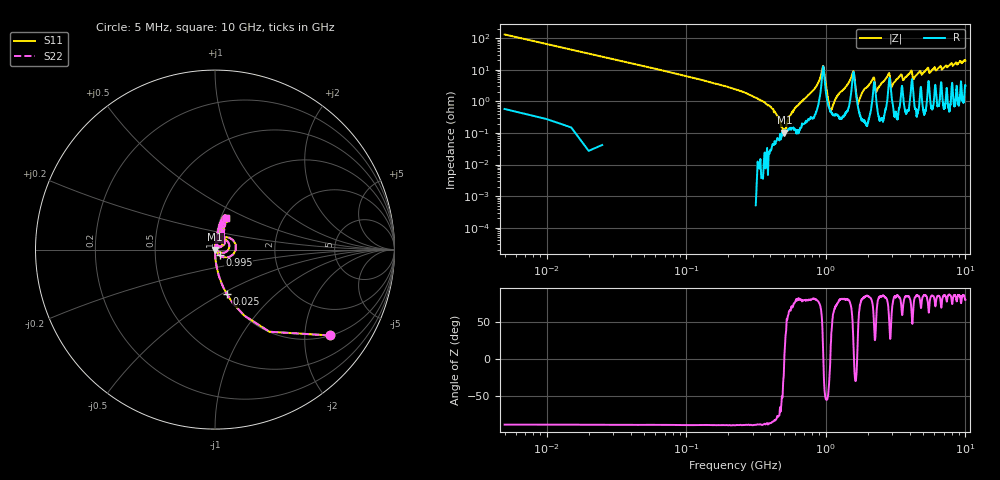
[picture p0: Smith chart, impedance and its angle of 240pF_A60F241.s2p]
! Amotech Co.,Ltd.
! http://www.amotech.co.kr/
! Part Number: A60F241
! These Parameters are Measured in Series Mode Connection
! Operation Temp=25[degC], DC Bias Voltage=0[V]
! Freq. Start=5[MHz] Stop=10[GHz], 2000[Steps]
! Date: Monday, July 20, 2020, 05:10:55
# GHZ S RI R 50.000000
!Freq.(Hz) S11(Real) S11(Imag) S21(Real) S21(Imag) S12(Real) S12(Imag) S22(Real) S22(Imag)
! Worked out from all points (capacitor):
!   2000 points, 5 MHz to 10 GHz, reference 50 ohm
!   read as one part in series: C = 240 pF near 55 MHz
!   lowest |Z| = 102 mohm at 505 MHz (marker M1)
!   series resonance near 504.3 MHz, so ESL is about 410 pH
!   S11 on the Smith chart (normalised r, x): 5 MHz: 1.01, -2.66; 25 MHz: 1.00, -0.53; 995 MHz: 1.05, -0.07; 10 GHz: 1.06, +0.39
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0.005  0.6384 -0.4783  0.3616 0.4783  0.3616 0.4783  0.6384 -0.4783
0.025  0.0655 -0.2467  0.9345 0.2467  0.9345 0.2467  0.0655 -0.2467
0.115  0.00261 -0.0545  0.9974 0.0545  0.9974 0.0545  0.00261 -0.0545
0.37  0.000151 -0.00869  0.9998 0.00869  0.9998 0.00869  0.000151 -0.00869
0.505  0.00102 7.58e-05  0.999 -7.58e-05  0.999 -7.58e-05  0.00102 7.58e-05
0.925  0.0306 0.0608  0.9694 -0.0608  0.9694 -0.0608  0.0306 0.0608
0.995  0.0253 -0.0318  0.9747 0.0318  0.9747 0.0318  0.0253 -0.0318
1.05  0.00682 -0.00581  0.9932 0.00581  0.9932 0.00581  0.00682 -0.00581
1.095  0.00439 0.0031  0.9956 -0.0031  0.9956 -0.0031  0.00439 0.0031
1.55  0.0463 0.0581  0.9537 -0.0581  0.9537 -0.0581  0.0463 0.0581
1.6  0.06 -0.0134  0.94 0.0134  0.94 0.0134  0.06 -0.0134
1.675  0.00998 -0.000486  0.99 0.000486  0.99 0.000486  0.00998 -0.000486
1.72  0.0055 0.00803  0.9945 -0.00803  0.9945 -0.00803  0.0055 0.00803
2.175  0.0191 0.0486  0.9809 -0.0486  0.9809 -0.0486  0.0191 0.0486
2.315  0.00855 0.0194  0.9914 -0.0194  0.9914 -0.0194  0.00855 0.0194
2.81  0.0309 0.0649  0.9691 -0.0649  0.9691 -0.0649  0.0309 0.0649
2.96  0.0143 0.024  0.9857 -0.024  0.9857 -0.024  0.0143 0.024
3.34  0.00948 0.058  0.9905 -0.058  0.9905 -0.058  0.00948 0.058
5.005  0.0117 0.0804  0.9883 -0.0804  0.9883 -0.0804  0.0117 0.0804
6.67  0.0488 0.1179  0.9512 -0.1179  0.9512 -0.1179  0.0488 0.1179
8.335  0.0293 0.1464  0.9707 -0.1464  0.9707 -0.1464  0.0293 0.1464
10  0.063 0.1754  0.937 -0.1754  0.937 -0.1754  0.063 0.1754
